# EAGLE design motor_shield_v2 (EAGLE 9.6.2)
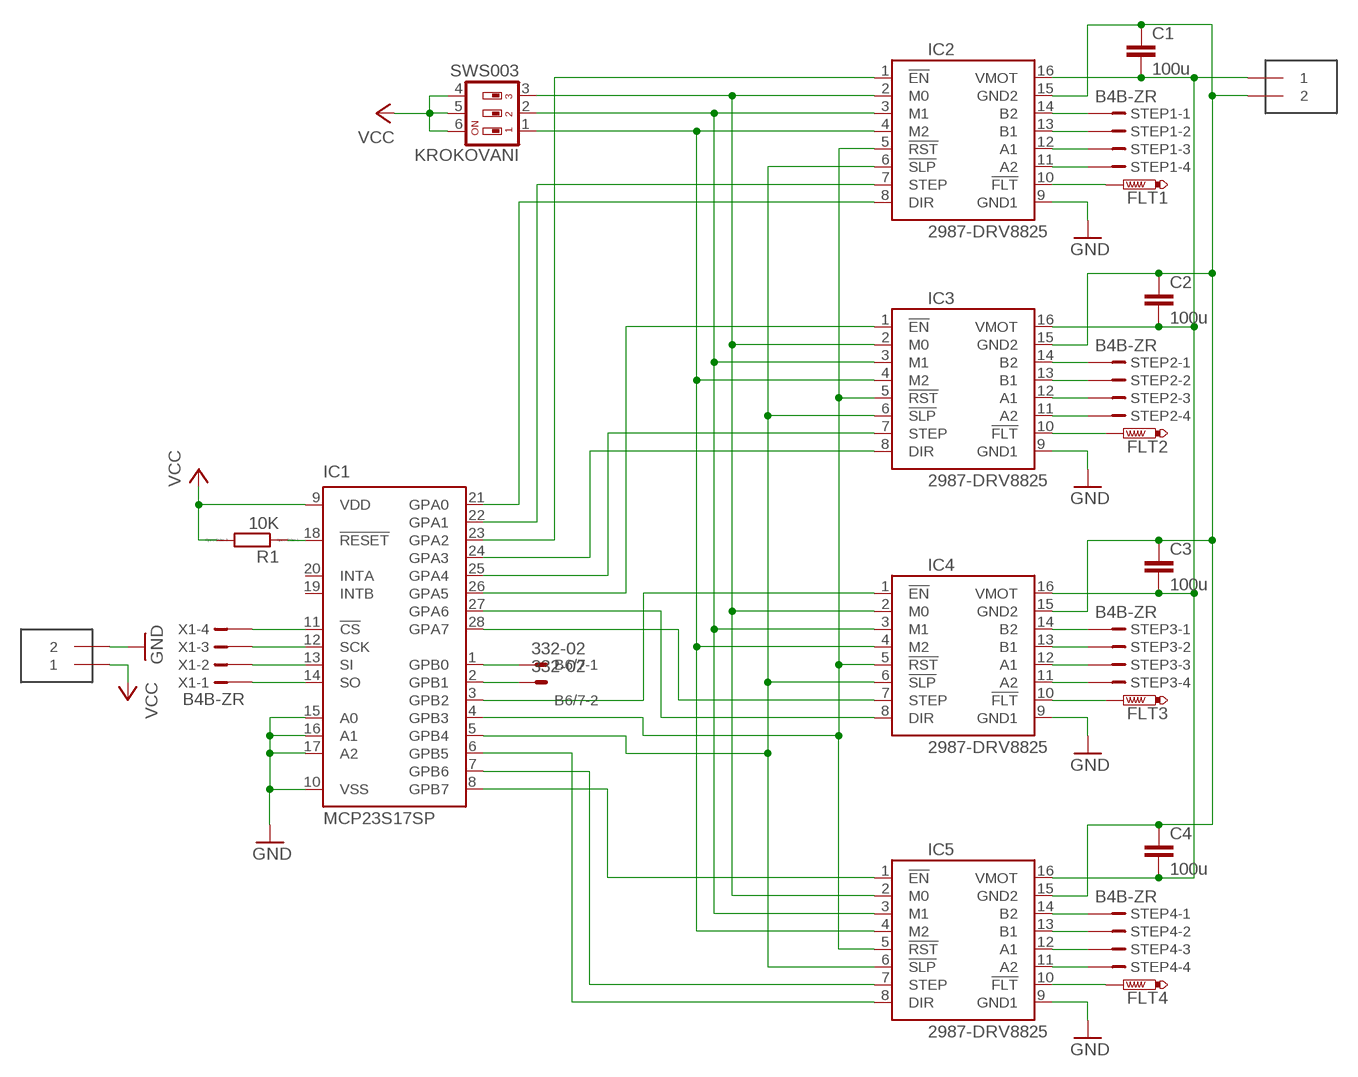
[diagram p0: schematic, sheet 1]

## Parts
B6/7  332-02  [332-02]
C1  100u  C-EU050-050X075  [C050-050X075]
C2  100u  C-EU050-050X075  [C050-050X075]
C3  100u  C-EU050-050X075  [C050-050X075]
C4  100u  C-EU050-050X075  [C050-050X075]
FLT1  PTR1B2,54  [B2,54]
FLT2  PTR1B2,54  [B2,54]
FLT3  PTR1B2,54  [B2,54]
FLT4  PTR1B2,54  [B2,54]
IC1  MCP23S17SP  [DIL28-3]
IC2  2987-DRV8825  [DRV8825]
IC3  2987-DRV8825  [DRV8825]
IC4  2987-DRV8825  [DRV8825]
IC5  2987-DRV8825  [DRV8825]
KROKOVANI  SWS003  [SMS-003]
R1  10K  RR0603  [R0603]
STEP1  B4B-ZR  [B4B-ZR]
STEP2  B4B-ZR  [B4B-ZR]
STEP3  B4B-ZR  [B4B-ZR]
STEP4  B4B-ZR  [B4B-ZR]
U$1  TERMINAL_2P  [KF301-2P]
U$2  TERMINAL_2P  [KF301-2P]
X1  B4B-ZR  [B4B-ZR]

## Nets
GND: IC1.10(VSS) IC1.15(A0) IC1.16(A1) IC1.17(A2) IC2.9(GND1) IC3.9(GND1) IC4.9(GND1) IC5.9(GND1) U$2.2
N$1: FLT4.TP IC5.10(!FLT)
N$2: FLT3.TP IC4.10(!FLT)
N$3: FLT2.TP IC3.10(!FLT)
N$4: IC1.24(GPA3) IC3.8(DIR)
N$5: IC1.28(GPA7) IC4.7(STEP)
N$6: FLT1.TP IC2.10(!FLT)
N$7: IC1.6(GPB5) IC5.8(DIR)
N$8: IC1.7(GPB6) IC5.7(STEP)
N$9: IC2.14(B2) STEP1.1
N$10: IC2.13(B1) STEP1.2
N$11: IC2.12(A1) STEP1.3
N$12: IC2.11(A2) STEP1.4
N$13: IC3.14(B2) STEP2.1
N$14: IC3.13(B1) STEP2.2
N$15: IC3.12(A1) STEP2.3
N$16: IC3.11(A2) STEP2.4
N$17: IC4.14(B2) STEP3.1
N$18: IC4.13(B1) STEP3.2
N$19: IC4.12(A1) STEP3.3
N$20: IC4.11(A2) STEP3.4
N$21: IC5.14(B2) STEP4.1
N$22: IC5.13(B1) STEP4.2
N$23: IC5.12(A1) STEP4.3
N$24: IC5.11(A2) STEP4.4
N$25: IC2.4(M2) IC3.4(M2) IC4.4(M2) IC5.4(M2) KROKOVANI.1
N$26: IC1.25(GPA4) IC3.7(STEP)
N$27: C1.2 C2.2 C3.2 C4.2 IC2.16(VMOT) IC3.16(VMOT) IC4.16(VMOT) IC5.16(VMOT) U$1.1
N$28: IC2.2(M0) IC3.2(M0) IC4.2(M0) IC5.2(M0) KROKOVANI.3
N$29: IC2.3(M1) IC3.3(M1) IC4.3(M1) IC5.3(M1) KROKOVANI.2
N$30: IC1.26(GPA5) IC3.1(!EN)
N$31: IC1.23(GPA2) IC2.1(!EN)
N$32: IC1.8(GPB7) IC5.1(!EN)
N$33: IC1.5(GPB4) IC2.6(!SLP) IC3.6(!SLP) IC4.6(!SLP) IC5.6(!SLP)
N$34: B6/7.1 IC1.1(GPB0)
N$35: IC1.4(GPB3) IC2.5(!RST) IC3.5(!RST) IC4.5(!RST) IC5.5(!RST)
N$36: IC1.11(!CS) X1.4
N$37: IC1.18(!RESET) R1.1
N$38: IC1.12(SCK) X1.3
N$39: IC1.13(SI) X1.2
N$40: IC1.14(SO) X1.1
N$41: B6/7.2 IC1.2(GPB1)
N$42: IC1.3(GPB2) IC4.1(!EN)
N$43: IC1.27(GPA6) IC4.8(DIR)
N$44: C1.1 C2.1 C3.1 C4.1 IC2.15(GND2) IC3.15(GND2) IC4.15(GND2) IC5.15(GND2) U$1.2
N$45: IC1.22(GPA1) IC2.7(STEP)
N$46: IC1.21(GPA0) IC2.8(DIR)
VCC: IC1.9(VDD) KROKOVANI.4 KROKOVANI.5 KROKOVANI.6 R1.2 U$2.1
Unconnected: IC1.19(INTB) IC1.20(INTA)

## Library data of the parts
B6/7 = con-garry:332-02: 2 Pin - 2mm Dual Row
C1-C4 = rcl:C-EU: CAPACITOR, European symbol; SPICEPREFIX: C
FLT1-FLT4 = testpad:PTR1: TEST PIN
IC1 = microchip:MCP23S17: http://ww1.microchip.com/downloads/en/DeviceDoc/21952a.pdf Source: http://ww1.microchip.com/downloads/en/DeviceDoc/21952a.pdf; MF: MICROCHIP; MPN: MCP23S17-E/SP; OC_FARNELL: 1292238; OC_NEWARK: 31K2951
IC2-IC5 = pololu-stepper-driver:2987-DRV8825: DRV8825 Stepper Motor Driver Carrier; High Current (Bulk; Header Pins Soldered) #2987 DRV8825 Stepper Motor Driver Carrier; High Current (Bulk; Header Pins Soldered) in Japan, Suzaku Lab. Ltd. #2987 DRV8825 大電流ステッピングモータドライバボード (バルク品 ピンヘッダ実装済み)
KROKOVANI = smd-special:SWS003: SMD Dip Switch 3 pol.
R1 = eagle-ltspice:R: RESISTOR, European symbol; SPICEMODEL: NONE; SPICEPREFIX: R
STEP1-STEP4 X1 = con-jst:?4B-ZR: ZH CONNECTOR 1.5 mm, 4 pin 1 row Source: http://www.jst.com .. eZH.pdf; MF: FARNELL; MPN: B4B-ZR(LF)(SN); OC_FARNELL: 1830916; OC_NEWARK: 37K9960
U$1 U$2 = KF301-2P-Terminal:TERMINAL_2P: Terminal Screw 2 Port 5mm Pitch

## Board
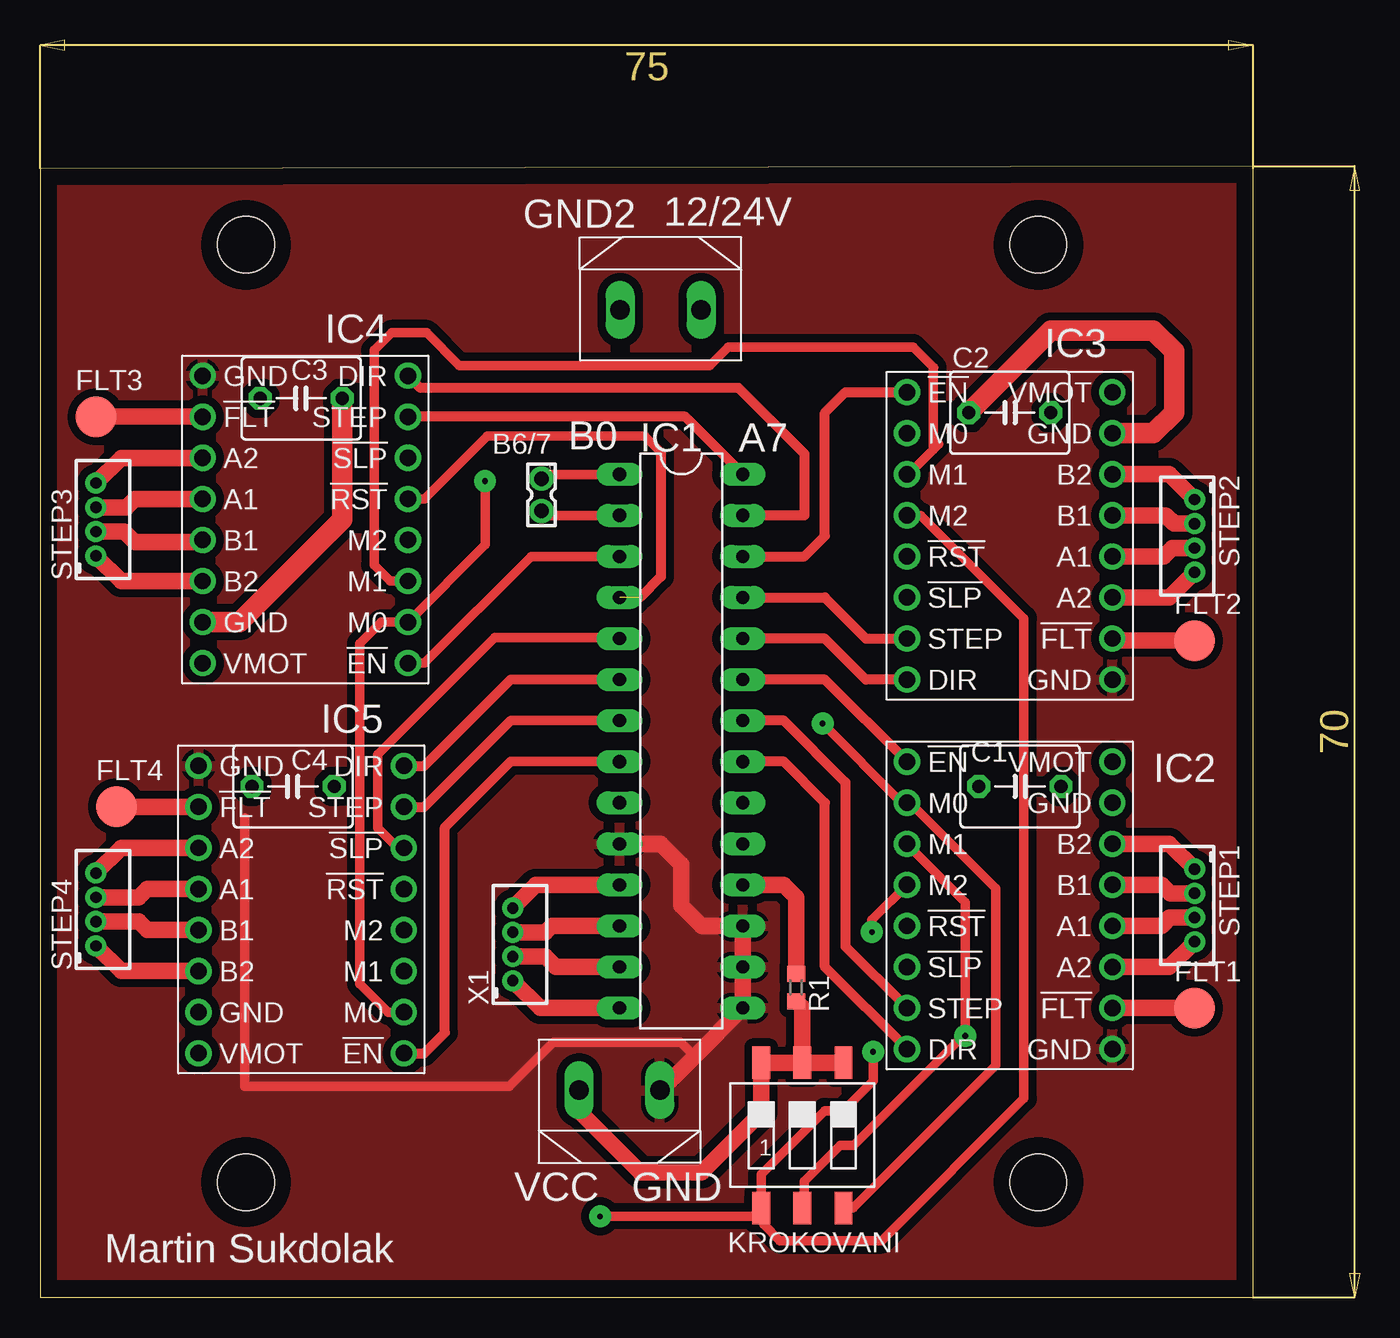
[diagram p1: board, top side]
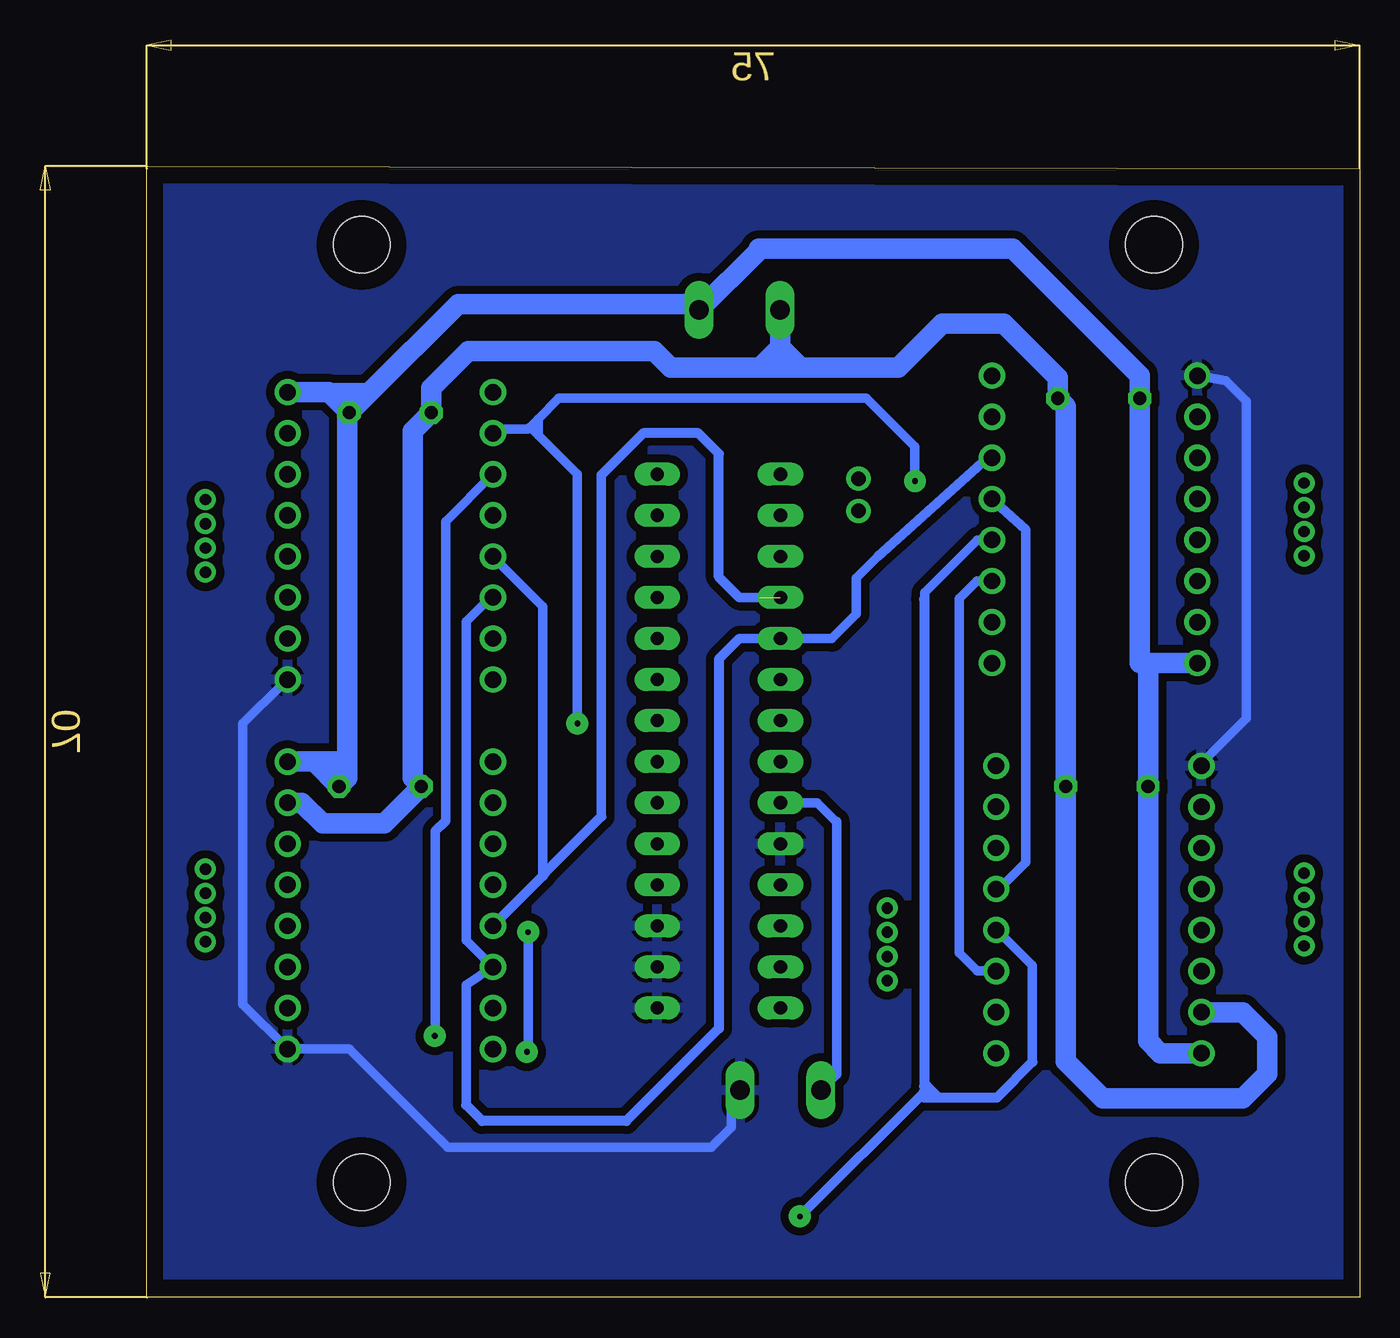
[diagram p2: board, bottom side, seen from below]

Size 81.58 x 77.77 mm. Coordinates in mm from the lower left corner, seen from the top.
Outline: 0,0 75,0 75,70 0,69.84 0,0
Copper layers (1*16): Top 0.035mm / dielectric 1.5mm / Bottom 0.035mm
Design rules "default *": minimum track width 0.6mm, minimum drill 0.35mm, track to track 0.5mm, track to pad 0.5mm, pad to pad 0.3mm, via to via 0.3mm, smd to smd 0.3mm, copper to edge 40mil, drill to drill 0.5mm, minimum pad ring 0.3mm, minimum via ring 0.5mm, stop-mask expansion 4mil, vias tented up to drill 0mil, thermal gap 10mil
Holes 3.5 mm at 12.71,7.13 12.71,65.13 61.71,65.13 61.71,7.13

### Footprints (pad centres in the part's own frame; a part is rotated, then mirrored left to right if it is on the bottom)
332-02 = drill 0.9 pad 1.27: 1 0,-1; 2 0,1
C050-050X075 = drill 0.813 octagon: 1 -2.54,0; 2 2.54,0
B2,54 = smd 2.54 x 2.54: TP 0,0
DIL28-3 = drill 0.813 long: 1 -16.51,-3.81; 2 -13.97,-3.81; 3 -11.43,-3.81; 4 -8.89,-3.81; 5 -6.35,-3.81; 6 -3.81,-3.81; 7 -1.27,-3.81; 8 1.27,-3.81; 9 3.81,-3.81; 10 6.35,-3.81; 11 8.89,-3.81; 12 11.43,-3.81; 13 13.97,-3.81; 14 16.51,-3.81; 15 16.51,3.81; 16 13.97,3.81; 17 11.43,3.81; 18 8.89,3.81; 19 6.35,3.81; 20 3.81,3.81; 21 1.27,3.81; 22 -1.27,3.81; 23 -3.81,3.81; 24 -6.35,3.81; 25 -8.89,3.81; 26 -11.43,3.81; 27 -13.97,3.81; 28 -16.51,3.81
DRV8825 = drill 1.016: 1 -6.35,8.89; 2 -6.35,6.35; 3 -6.35,3.81; 4 -6.35,1.27; 5 -6.35,-1.27; 6 -6.35,-3.81; 7 -6.35,-6.35; 8 -6.35,-8.89; 9 6.35,-8.89; 10 6.35,-6.35; 11 6.35,-3.81; 12 6.35,-1.27; 13 6.35,1.27; 14 6.35,3.81; 15 6.35,6.35; 16 6.35,8.89
SMS-003 = smd 1.092 x 2.007: 1 -2.54,-4.496; 2 0,-4.496; 3 2.54,-4.496; 4 2.54,4.496; 5 0,4.496; 6 -2.54,4.496
R0603 = smd 1 x 1.1: 1 -0.85,0; 2 0.85,0
B4B-ZR = drill 0.7 pad 1.1: 1 -2.25,0; 2 -0.75,0; 3 0.75,0; 4 2.25,0
KF301-2P = drill 1.2 pad 1.778 long: 1 -2.5,0; 2 2.5,0

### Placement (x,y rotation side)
B6/7  30.99,49.66 180 top
C1  60.58,31.62 0 top
C2  59.94,54.74 0 top
C3  16.13,55.63 180 top
C4  15.62,31.62 180 top
FLT1  71.37,17.91 0 top
FLT2  71.37,40.64 0 top
FLT3  3.43,54.48 0 top
FLT4  4.7,30.35 0 top
IC1  39.62,34.42 270 top
IC2  59.94,24.26 0 top
IC3  59.94,47.12 0 top
IC4  16.38,48.13 180 top
IC5  16.13,24 180 top
KROKOVANI  47.12,10.03 0 top
R1  46.74,19.18 270 top
STEP1  71.37,24.26 270 top
STEP2  71.37,47.12 270 top
STEP3  3.43,48.13 90 top
STEP4  3.43,24 90 top
U$1  38.35,61.09 180 top
U$2  35.81,12.83 0 top
X1  29.21,21.84 90 top

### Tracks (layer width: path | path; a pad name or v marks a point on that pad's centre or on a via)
GND
  Top 0.6: 12.65,29.66 12.65,13.05 29,13.05 31.73,15.79 39.61,15.79 40.46,14.93 | 10,32.81 IC5.9
  Top 1.016: U$2.2 38.35,12.83 40.46,14.93 IC1.15 IC1.16 IC1.17 40.89,22.99 39.62,24.26 39.62,26.8 38.35,28.07 IC1.10
  Bottom 0.6: IC4.9 8.26,56.73 7,55.46 7,35.81 9.75,33.06 IC5.9 | IC3.9 66.53,38.03 69.05,35.51 69.05,18.13 IC2.9 62.48,15.37 56.4,9.29 40.11,9.29 38.86,10.53 38.86,12.28 U$2.2
  pour Top: 0.25,68.71 0.25,1.4 75.82,1.4 75.82,68.71
  pour Bottom: 0.25,68.71 0.25,1.4 75.82,1.4 75.82,1.4 75.82,68.71
N$1
  Top 1.016: FLT4.TP IC5.10
N$2
  Top 1.016: FLT3.TP IC4.10
N$3
  Top 1.016: FLT2.TP 66.42,40.64 IC3.10
N$4
  Top 0.61: IC3.8 51.05,38.23 48.51,40.77 IC1.24
N$5
  Top 0.61: IC4.7 39.88,54.48 IC1.28
N$6
  Top 1.016: FLT1.TP IC2.10
N$7
  Top 0.6: 29.08,38.23 IC1.6
  Top 0.61: IC5.8 23.75,32.89 29.08,38.23
N$8
  Top 0.6: 29.05,35.65 29.08,35.69 IC1.7
  Top 0.61: IC5.7 23.75,30.35 29.05,35.65
N$9
  Top 1.016: IC2.14 69.81,28.07 STEP1.1
N$10
  Top 1.016: IC2.13 69.34,25.53 69.86,25.01 STEP1.2
N$11
  Top 1.016: IC2.12 66.31,23 69.34,23 69.85,23.51 STEP1.3
N$12
  Top 1.016: STEP1.4 69.81,20.45 IC2.11
N$13
  Top 1.016: IC3.14 69.81,50.93 STEP2.1
N$14
  Top 1.016: IC3.13 69.6,48.39 70.12,47.87 STEP2.2
N$15
  Top 1.016: IC3.12 69.47,45.85 69.99,46.37 STEP2.3
N$16
  Top 1.016: STEP2.4 69.81,43.31 IC3.11
N$17
  Top 1.016: STEP3.1 4.99,44.32 IC4.14
N$18
  Top 1.016: STEP3.2 5.2,47.38 5.84,46.74 9.91,46.74 IC4.13
N$19
  Top 1.016: STEP3.3 5.32,48.88 5.84,49.4 IC4.12
N$20
  Top 1.016: STEP3.4 4.99,51.94 IC4.11
N$21
  Top 1.016: STEP4.1 4.99,20.19 IC5.14
N$22
  Top 1.016: IC5.13 6.6,22.73 6.08,23.25 STEP4.2
N$23
  Top 1.016: IC5.12 6.6,25.27 6.08,24.75 STEP4.3
N$24
  Top 1.016: STEP4.4 4.99,27.81 IC5.11
N$25  (via drill 0.35)
  Top 0.6: KROKOVANI.1 44.05,5.01 v34.61,5.01 | IC2.4 51.42,23.35 v51.42,22.61 | 44.33,6.12 KROKOVANI.1 | IC3.4 54.44,48.39 60.82,42.02 60.82,12.31 52.03,3.52 45.73,3.52 44.72,4.54 KROKOVANI.1 | KROKOVANI.1 44.58,7.62 48.51,11.56 49.66,11.56 51.5,13.4 v51.5,15.19
  Bottom 0.6: 20.24,14.56 20.24,20.55 22.25,22.56 IC5.4 | v51.5,15.19 51.42,15.27 v51.42,22.61 | 26.9,43.22 26.9,43.6 23.64,46.86 IC4.4 | 26.04,12.38 26.73,13.08 26.92,13.08
  Bottom 0.61: 20.24,14.56 22.42,12.38 26.04,12.38 26.92,12.38 26.92,12.63 | 26.92,12.63 26.99,12.63 v34.61,5.01 | 26.9,43.22 26.92,43.2 26.92,13.08 26.92,12.63
N$26
  Top 0.61: IC1.25 48.51,43.31 51.05,40.77 IC3.7
N$27
  Bottom 1.27: IC2.16 64.64,33.15 | 64.64,33.15 C1.2 62.61,32.13 62.61,33.4 | 62.61,33.4 62.61,54.61 C2.2 | C2.2 63.69,55.94 | IC3.16 63.75,56.01 63.69,55.94 | C2.2 61.28,55.94 | 61.28,55.94 55.75,61.47 41.23,61.47 U$1.1 37.17,64.77 37.17,64.9 21.46,64.9 13.59,57.02 C3.2 13.59,39.24 13.08,39.24 | IC4.16 13.08,39.24 | IC5.16 12.32,15.11 13.08,15.88 C4.2 13.08,39.24 | 64.64,33.15 62.87,33.15 62.61,33.4 | 61.28,55.94 63.69,55.94
N$28  (via drill 0.35)
  Top 0.6: IC5.2 21.51,17.65 19.75,19.42 19.75,40.46 21.07,41.78 IC4.2 | KROKOVANI.3 50.26,5.54 59.07,14.35 59.07,25.32 53.78,30.61 IC2.2 53.28,30.61 v48.38,35.51 | IC4.2 22.84,41.78 | IC4.2 27.52,46.57 27.5,46.57 v27.5,50.51
  Bottom 0.6: v48.38,35.51 48.38,50.93 50.8,53.35 | 27.37,50.63 v27.5,50.51 27.5,52.65 30.5,55.64 49.51,55.64 50.8,54.36 | IC3.2 53.34,53.72 51.44,53.72 51.3,53.85 | 51.3,53.85 50.8,53.35 | 50.8,54.36 51.3,53.85 | 50.8,54.36 50.8,53.35
N$29  (via drill 0.35)
  Top 0.6: KROKOVANI.2 47.24,5.65 47.24,7.17 49.48,9.41 50.3,9.41 57.07,16.18 v57.19,16.18 57.19,24.45 53.78,27.86 IC2.3 | 55.23,52.47 53.78,51.03 IC3.3 | 55.23,52.47 55.54,52.78 | IC4.3 21.64,44.32 20.64,45.32 20.64,58.6 21.73,59.69 23.88,59.69 25.91,57.66 41.4,57.66 42.55,58.8 53.98,58.8 55.24,57.53 55.23,57.51 55.23,52.47
  Bottom 0.6: IC5.3 23.65,20.19 24.76,21.3 24.76,43.24 23.68,44.32 IC4.3 | v57.19,16.18 57.15,16.23 57.15,28.86 56.52,29.49 56.52,48.01 IC3.3
N$30
  Top 0.61: IC1.26 47.24,45.85 48.51,47.12 48.51,54.74 49.78,56.01 IC3.1
N$31
  Top 0.61: IC1.23 48.51,38.23 IC2.1
N$32
  Top 0.6: 29.08,33.15 IC1.8
  Top 0.61: IC5.1 23.75,15.11 25.02,16.38 25.02,29.08 29.08,33.15
N$33
  Top 0.6: IC5.6 22.11,27.81 20.87,29.05 20.87,33.6 28.09,40.82 35.76,40.82 IC1.5
  Bottom 0.6: IC3.6 53.78,43.28 55.24,41.82 55.24,22.1 IC2.6 55.25,19.34 55.25,11.92 | IC4.6 23.02,51.94 29.79,45.85 31.11,44.52 31.11,42.29 32.64,40.77 IC1.5 38.35,40.77
  Bottom 0.61: 55.25,11.92 54.26,10.92 45.34,10.92 39.62,16.64 39.62,39.5 38.35,40.77
N$34
  Top 0.6: IC1.1 35.8,50.91 31.24,50.91 B6/7.1
N$35  (1 unrouted)
  Top 0.6: 38.37,52.29 37.38,53.28 27.62,53.28 23.75,49.4 IC4.5
  Top 0.61: 38.37,52.29 38.37,44.59 37.08,43.31
  Bottom 0.6: 50.51,26.26 50.51,42.75 53.53,45.78 IC3.5 | IC5.5 22.25,25.31 20.64,26.92 20.64,47.51 IC4.5 | 46.88,50.89 46.88,29.76 | 38.35,43.31 IC1.4
  Bottom 0.61: 38.35,43.31 39.62,44.58 39.62,52.2 40.89,53.47 44.31,53.47 46.88,50.89 | 46.88,29.76 50.38,26.26 50.51,26.26 50.51,26.07 IC2.5
N$36
  Top 1.016: X1.4 30.64,25.53 IC1.11
N$37
  Top 1.016: R1.1 46.74,24.77 45.97,25.53 IC1.18
N$38
  Top 1.016: X1.3 31.23,22.59 31.62,22.99 IC1.12
N$39
  Top 1.016: IC1.13 31.88,20.45 31.23,21.09 X1.2
N$40
  Top 1.016: IC1.14 30.9,17.91 X1.1
N$41
  Top 0.6: IC1.2 31.26,48.39 B6/7.2
N$42
  Top 0.6: IC4.1 23.75,39.24 30.35,45.85 IC1.3
  Top 0.61: IC4.1 22.86,39.24
N$43
  Top 0.61: IC4.8 23.5,56.26 43.18,56.26 47.24,52.2 47.24,48.39 IC1.27
N$44
  Top 1.27: IC4.15 12.32,41.78 18.67,48.13 C3.1 | IC3.15 68.83,53.47 70.1,54.74 70.1,58.55 68.83,59.82 62.48,59.82 C2.1
  Bottom 1.27: IC2.15 65.41,30.61 64.14,29.34 60.33,29.34 C1.1 58.55,32.13 58.55,53.59 C2.1 57.4,56.26 55.12,58.55 43.62,58.55 42.6,57.53 37.08,57.53 | U$1.2 35.85,61.05 35.81,61.01 35.81,58.8 | IC5.15 7.24,17.65 5.71,16.13 5.71,13.84 7.24,12.32 15.88,12.32 18.16,14.61 C4.1 18.16,55.12 C3.1 18.67,56.9 22.01,60.24 25.82,60.24 28.53,57.53 34.54,57.53 | 37.08,57.53 35.81,57.53 | 35.81,57.53 35.81,58.8 | 35.81,57.53 34.54,57.53 | 34.54,57.53 35.81,58.8 | 35.81,58.8 37.08,57.53
N$45
  Top 0.61: IC2.7 49.78,21.72 49.78,31.88 45.97,35.69 IC1.22
N$46
  Top 0.61: IC2.8 48.51,20.45 48.51,30.61 45.97,33.15 IC1.21
VCC
  Top 1.016: U$2.1 33.31,11.52 37.08,7.75 40.89,7.75 44.58,11.43 KROKOVANI.6 KROKOVANI.5 | KROKOVANI.5 KROKOVANI.4 | R1.2 47.12,17.95 KROKOVANI.5
  Bottom 0.6: U$2.1 32.35,13.79 32.35,29.46 32.38,29.46 33.53,30.61 IC1.9

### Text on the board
tPlace: GND2 | 12/24V | B0 | A7 | VCC | GND | Martin Sukdolak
